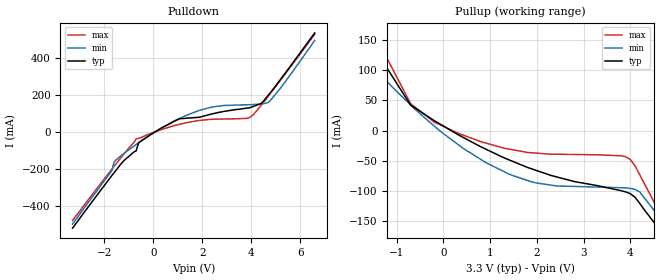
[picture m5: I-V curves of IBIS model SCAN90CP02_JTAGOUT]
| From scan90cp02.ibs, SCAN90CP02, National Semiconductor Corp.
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[Model]   SCAN90CP02_JTAGOUT
Model_type Output
Polarity Non-Inverting
Vref=0.0
Vmeas=1.65
Rref=500
Cref=50p
C_comp   5pF   5pF   5pF
[Temperature Range] 25   85   -40
[Voltage Range]   3.3   3.0   3.6
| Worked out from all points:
|   slope of the pulldown table from 0 to 0.495 V, typ, clamps not added: 12.9 ohm
|   slope of the pullup table from 0 to 0.495 V, typ, clamps not added: 22.7 ohm
[Pullup]
|Vtable   I(typ)   I(min)   I(max)
-3.3V     539mA      495mA      529mA
-1.7V     187mA      202mA      200mA
-1.5V     153mA      170mA      168mA
-1.4V     137mA      159mA      151mA
-1.3V     120mA      89.1mA     135mA
-700mV    42mA       42.5mA     44.5mA
300mV     -6.33mA    -22.5mA    -4.05mA
1.4V      -48.6mA    -72.3mA    -30.8mA
3.9V      -102mA     -95.3mA    -43.6mA
4.2V      -121mA     -102mA     -73.5mA
4.8V      -200mA     -172mA     -167mA
6.6V      -516mA     -495mA     -476mA
[Pulldown]
|V(pulldown)   I(typ)   I(min)   I(max)
-3.3V     -518mA     -496mA     -477mA
-1.7V     -235mA     -210mA     -201mA
-1.6V     -219mA     -161mA     -184mA
-1.2V     -154mA     -115mA     -118mA
-700mV    -101mA     -66.9mA    -36.2mA
-600mV    -57.4mA    -57.4mA    -33.7mA
1.1V      72.9mA     74.9mA     42.8mA
2.4V      98.3mA     135mA      69mA
4V        134mA      148mA      83.9mA
4.4V      154mA      151mA      143mA
4.8V      215mA      173mA      211mA
6.6V      535mA      495mA      528mA
[Ramp]
|   typ   min   max
dV/dt_r   1.26V/.185ns   1.5V/.060ns   0.96V/.200ns
dV/dt_f   1.45V/.240ns   1.64V/.12ns   1.15V/.260ns
R_load=50
|[End   SCAN90CP02_JTAGOUT
